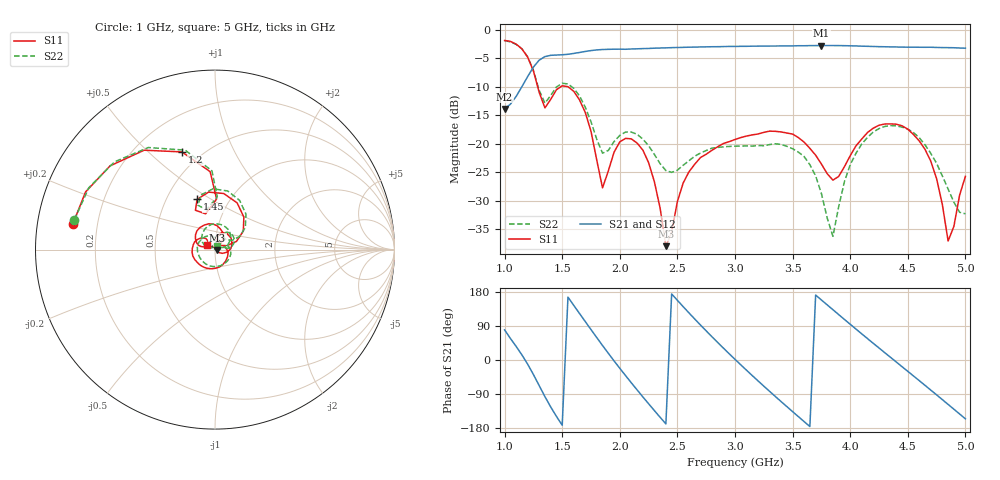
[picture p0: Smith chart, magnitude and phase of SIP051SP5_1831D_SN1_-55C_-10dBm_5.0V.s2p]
# GHz  S  dB  R  50
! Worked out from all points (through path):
!   81 points, 1 GHz to 5 GHz, reference 50 ohm
!   highest |S21| = -2.77 dB at 3.75 GHz (marker M1); lowest = -13.9 dB at 1 GHz (marker M2)
!   lowest |S11| = -38.0 dB at 2.4 GHz (marker M3), VSWR 1.03, Z = 51.2 - j0.353 ohm
!   |S11| at or under -10 dB: 1.287 GHz to 1.488 GHz (201.4 MHz wide, 14.5 % of centre); 1.55 GHz to end of sweep
!   |S22| runs from -36.3 to -1.9 dB; largest |S21 - S12| = 0.0024
!   S11 on the Smith chart (normalised r, x): 1 GHz: 0.11, +0.09; 1.2 GHz: 0.39, +0.64; 1.45 GHz: 0.71, +0.43; 5 GHz: 0.91, +0.05
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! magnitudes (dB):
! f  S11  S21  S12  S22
! 1 GHz  -1.9  -13.9  -13.9  -1.9
! 1.2 GHz  -4.8  -8.2  -8.2  -4.8
! 1.35 GHz  -13.7  -4.7  -4.7  -12.9
! 1.45 GHz  -10.5  -4.4  -4.4  -10.0
! 1.7 GHz  -14.5  -3.8  -3.8  -13.6
! 1.85 GHz  -27.8  -3.5  -3.5  -21.7
! 2 GHz  -19.7  -3.4  -3.4  -18.5
! 2.1 GHz  -19.2  -3.4  -3.4  -18.0
! 2.25 GHz  -23.3  -3.3  -3.3  -20.4
! 2.35 GHz  -31.3  -3.2  -3.2  -23.5
! 2.4 GHz  -38.0  -3.2  -3.2  -24.7
! 2.6 GHz  -24.9  -3.1  -3.1  -23.0
! 3 GHz  -19.3  -2.9  -2.9  -20.4
! 3.45 GHz  -18.1  -2.9  -2.8  -20.5
! 3.7 GHz  -22.0  -2.8  -2.8  -25.6
! 3.75 GHz  -23.6  -2.8  -2.8  -28.7
! 3.85 GHz  -26.4  -2.8  -2.8  -36.3
! 4.05 GHz  -20.4  -2.8  -2.9  -21.7
! 4.35 GHz  -16.5  -3.0  -3.0  -16.8
! 4.65 GHz  -21.0  -3.1  -3.1  -20.2
! 4.85 GHz  -37.1  -3.1  -3.2  -28.0
! 5 GHz  -25.7  -3.2  -3.3  -32.3
